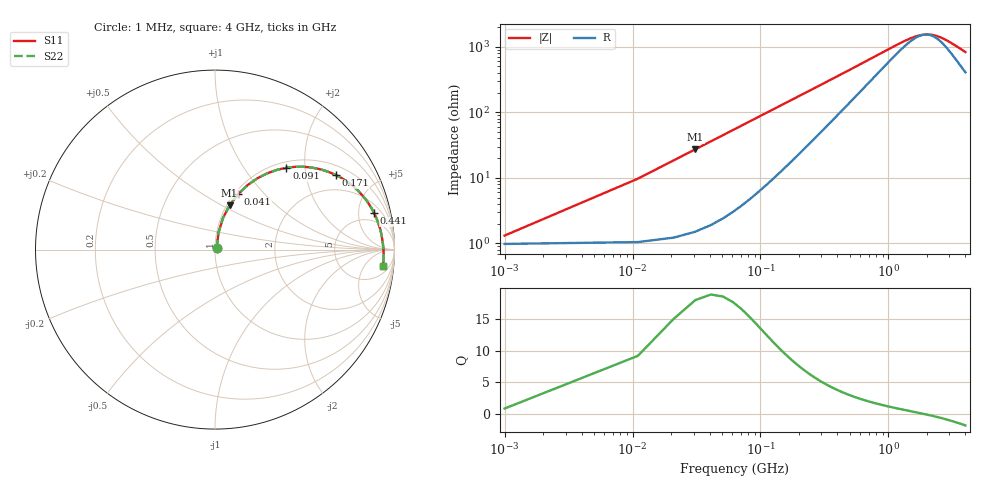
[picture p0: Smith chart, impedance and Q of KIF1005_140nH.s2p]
!version-2
!date-12.2020
!Series
# MHz S RI R 50
!Freq ReS11 ImS11 ReS21 ImS21 ReS12 ImS12 ReS22 ImS22
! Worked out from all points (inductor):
!   401 points, 1 MHz to 4 GHz, reference 50 ohm
!   read as one part in series: L = 140 nH near 21 MHz
!   highest Q = 16.6 at 31 MHz (marker M1), where L = 140 nH
!   self-resonance near 1.935 GHz
!   S11 on the Smith chart (normalised r, x): 1 MHz: 1.02, +0.02; 41 MHz: 1.04, +0.72; 91 MHz: 1.11, +1.60; 171 MHz: 1.34, +2.99; 441 MHz: 3.19, +7.52; 4 GHz: 9, -14
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1  0.00983 0.00862  0.9902 -0.00862  0.9902 -0.00862  0.00983 0.00862
11  0.0194 0.0938  0.9806 -0.0938  0.9806 -0.0938  0.0194 0.0938
31  0.081 0.2465  0.919 -0.2465  0.919 -0.2465  0.081 0.2465
41  0.1277 0.3083  0.8723 -0.3083  0.8723 -0.3083  0.1277 0.3083
51  0.1804 0.3584  0.8196 -0.3584  0.8196 -0.3584  0.1804 0.3584
61  0.2359 0.3972  0.7641 -0.3972  0.7641 -0.3972  0.2359 0.3972
91  0.3975 0.4559  0.6025 -0.4559  0.6025 -0.4559  0.3975 0.4559
131  0.5648 0.4524  0.4352 -0.4524  0.4352 -0.4524  0.5648 0.4524
171  0.6755 0.4144  0.3245 -0.4144  0.3245 -0.4144  0.6755 0.4144
221  0.761 0.36  0.239 -0.36  0.239 -0.36  0.761 0.36
271  0.8125 0.3118  0.1875 -0.3118  0.1875 -0.3118  0.8125 0.3118
341  0.8549 0.258  0.1451 -0.258  0.1451 -0.258  0.8549 0.258
441  0.8869 0.2029  0.1131 -0.2029  0.1131 -0.2029  0.8869 0.2029
671  0.916 0.1285  0.084 -0.1285  0.084 -0.1285  0.916 0.1285
981  0.9288 0.0759  0.0712 -0.0759  0.0712 -0.0759  0.9288 0.0759
1341  0.9346 0.0396  0.0654 -0.0396  0.0654 -0.0396  0.9346 0.0396
1671  0.9373 0.0158  0.0627 -0.0158  0.0627 -0.0158  0.9373 0.0158
2001  0.9389 -0.00367  0.0611 0.00367  0.0611 0.00367  0.9389 -0.00367
2301  0.9397 -0.0193  0.0603 0.0193  0.0603 0.0193  0.9397 -0.0193
2671  0.94 -0.0369  0.06 0.0369  0.06 0.0369  0.94 -0.0369
3341  0.9386 -0.0662  0.0614 0.0662  0.0614 0.0662  0.9386 -0.0662
4000  0.9348 -0.0928  0.0652 0.0928  0.0652 0.0928  0.9348 -0.0928
